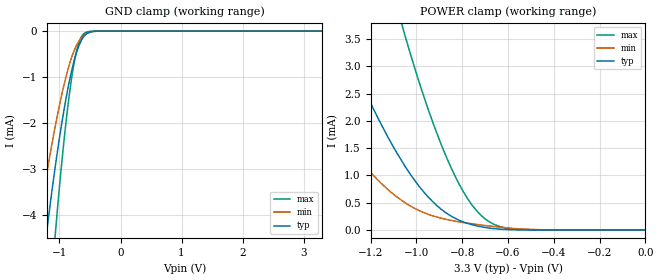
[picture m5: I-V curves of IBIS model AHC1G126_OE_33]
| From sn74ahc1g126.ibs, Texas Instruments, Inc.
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[Model]   AHC1G126_OE_33
Model_type  Input
Vinl=0.9
Vinh=2.1
| variable   typ   min   max
C_comp   2.80pF   2.37pF   3.01pF
[Temperature Range]   40   100   -40
| Ambient temperature   25   85   -40
[Voltage range]   3.3   3   3.6
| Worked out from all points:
|   GND clamp passes 1 mA (typ) near -0.82 V on its own axis
|   POWER clamp passes 1 mA (typ) near -1.02 V on its own axis
[GND Clamp]
| AHC1G126_OE_33
|   Voltage   I(typ)   I(min)   I(max)
-3.3V     -41.29mA   -27.62mA   -63.42mA
-1.365V   -6.183mA   -4.403mA   -9.863mA
-1.35V    -6mA       -4.273mA   -9.556mA
-1.2V     -4.277mA   -3.039mA   -6.665mA
-1.065V   -2.914mA   -2.046mA   -4.374mA
-905mV    -1.561mA   -1.059mA   -2.131mA
-785mV    -781.4uA   -515.6uA   -891.6uA
-735mV    -531.9uA   -353.2uA   -522.8uA
-675mV    -299.9uA   -209.3uA   -225.4uA
-560mV    -61.62uA   -59.85uA   -23.23uA
-305mV    -378nA     -548.6nA   -22.17nA
3.3V      168pA      26.63nA    3.503pA
[POWER Clamp]
| AHC1G126_OE_33
|   Voltage   I(typ)   I(min)   I(max)
-3.3V     39.15mA    24.34mA    67.14mA
-1.615V   6.939mA    3.73mA     14.64mA
-1.365V   3.941mA    1.959mA    9.109mA
-1.325V   3.522mA    1.718mA    8.31mA
-1.085V   1.412mA    605.2uA    4.092mA
-1.05V    1.172mA    501.4uA    3.571mA
-945mV    589.1uA    283.5uA    2.172mA
-845mV    246.5uA    172.8uA    1.111mA
-780mV    125uA      126.8uA    598.2uA
-700mV    46.04uA    82.19uA    203.1uA
-550mV    1.827uA    19.73uA    9.061uA
-48.03fV  168pA      645.8pA    4.332pA
